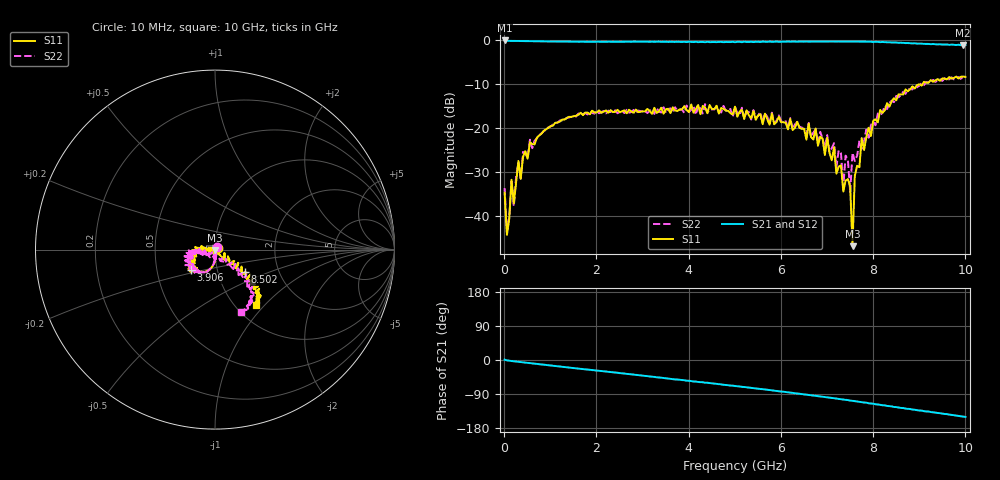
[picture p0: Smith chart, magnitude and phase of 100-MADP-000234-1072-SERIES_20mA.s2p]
!Agilent Technologies,E8364C,MY48140145,A.09.42.15
!Agilent E8364C: A.09.42.15
!Date: Wednesday, December 02, 2020 08:32:05
!Correction: S11(Full 2 Port(1,2))
!S21(Full 2 Port(1,2))
!S12(Full 2 Port(1,2))
!S22(Full 2 Port(1,2))
!S2P File: Measurements: S11, S21, S12, S22:
# Hz S  dB  R 50
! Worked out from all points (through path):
!   201 points, 10 MHz to 10 GHz, reference 50 ohm
!   highest |S21| = -0.03 dB at 10 MHz (marker M1); lowest = -1.1 dB at 9.95 GHz (marker M2)
!   group delay of S21, straight-line fit = 41 ps
!   lowest |S11| = -47.0 dB at 7.552 GHz (marker M3), VSWR 1.01, Z = 49.8 - j0.39 ohm
!   |S11| at or under -10 dB: start of sweep to 9.071 GHz
!   |S22| runs from -43.8 to -8.2 dB; largest |S21 - S12| = 0.022
!   S11 on the Smith chart (normalised r, x): 10 MHz: 1.03, +0.02; 3.906 GHz: 0.74, -0.17; 8.502 GHz: 1.34, -0.35; 10 GHz: 1.23, -0.89
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1e7  -34.74 36.7  -0.03 0.9  -0.04 -0.3  -33.71 50.2
5.995e7  -44.41 -53.2  -0.11 -1.0  -0.12 -1.1  -43.79 -65.9
1.5985e8  -31.82 -75.7  -0.13 -2.7  -0.12 -2.7  -32.09 -73.4
2.098e8  -37.22 -64.2  -0.14 -3.4  -0.13 -3.5  -37.87 -75.0
3.097e8  -27.52 -84.9  -0.16 -4.9  -0.16 -4.9  -27.92 -80.5
5.5945e8  -23.23 -92.7  -0.20 -8.5  -0.20 -8.5  -22.68 -89.9
1.7083e9  -17.07 -118.5  -0.33 -24.0  -0.31 -23.8  -16.87 -117.2
3.35665e9  -16.19 -137.2  -0.31 -46.0  -0.33 -46.2  -16.28 -126.9
3.9061e9  -15.00 -140.1  -0.35 -53.4  -0.35 -54.0  -16.59 -135.2
5.005e9  -15.15 -150.6  -0.44 -68.7  -0.41 -68.6  -15.17 -167.8
6.7033e9  -22.63 173.6  -0.27 -93.9  -0.24 -93.5  -21.08 176.7
7.3027e9  -28.53 -171.8  -0.30 -103.4  -0.28 -103.8  -25.77 -123.7
7.35265e9  -34.51 -99.4  -0.28 -104.4  -0.25 -104.0  -33.53 -137.8
7.45255e9  -31.66 -108.2  -0.28 -105.7  -0.27 -106.1  -27.26 -87.4
7.5025e9  -33.33 -50.9  -0.28 -107.1  -0.25 -106.6  -34.59 -111.7
7.55245e9  -46.97 -119.1  -0.28 -107.7  -0.30 -108.0  -25.67 -95.8
7.6024e9  -30.92 -50.3  -0.28 -108.6  -0.27 -108.6  -27.55 -74.6
7.75225e9  -22.31 -45.8  -0.32 -111.3  -0.28 -110.9  -24.79 -40.9
8.35165e9  -15.12 -32.6  -0.45 -121.9  -0.46 -121.9  -14.26 -47.3
8.5015e9  -13.69 -36.9  -0.50 -124.3  -0.53 -124.7  -12.68 -45.3
9.95005e9  -8.28 -51.0  -1.10 -149.5  -1.12 -149.3  -8.25 -67.6
1e10  -8.33 -53.7  -1.08 -150.3  -1.09 -150.3  -8.45 -67.2
